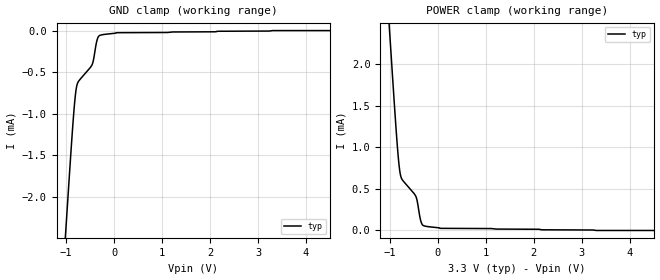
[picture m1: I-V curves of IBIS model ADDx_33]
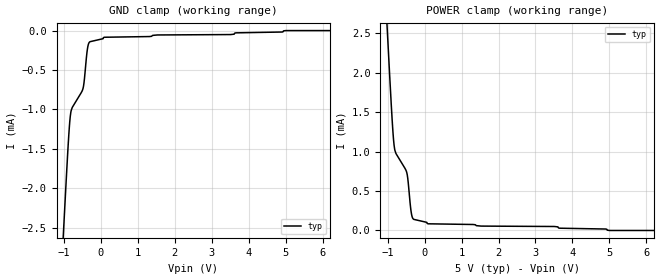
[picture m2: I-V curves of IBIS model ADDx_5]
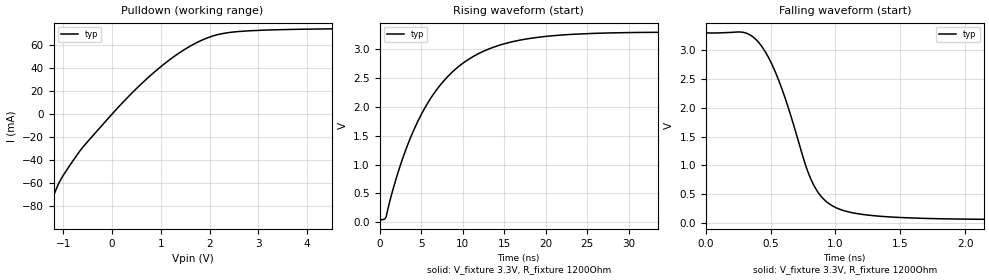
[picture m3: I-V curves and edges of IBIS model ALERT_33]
|Texas Instruments Incorporated
|Digital Temperature Sensor
|   with I2C Interface
| Marketing part#   Digital Voltage Range   Package-type   #pins
|TMP101NA/250   2.7 to 5.5   SOT   6
|TMP101NA/250G4   2.7 to 5.5   SOT   6
|TMP101NA/3K   2.7 to 5.5   SOT   6
|TMP101NA/3KG4   2.7 to 5.5   SOT   6
[IBIS Ver]   4.0
[File name]   tmp101.ibs
[File Rev]   1.0
[Date]   12/16/2010
[Source]   Texas Instruments Incorporated.
   Analog-eLab, HPA
   12500 TI Blvd
   Dallas, TX -75243
   For Support e-mail: elab_ibis@list.ti.com
[Notes]   Revision History:
   1.0: 12/16/2010
   - Model only contains nominal corner (27 degC, nominal
   process) for supply voltages of 3.3V and 5V.
   - Initial version of the model
   - Initial Model generated from simulations in TIspiceD
   - Model names with a trailing _33 contains the model for
   3.3V (3V and 3.6V). Model names with trailing _5 contains
   the model for 5V (4.5V and 5.5V) operation.
   - Model not matched to measurements
   - C_comp although listed in numerical order of value are
   obtained from varying PVT conditions. For PVT conditions
   for each specific value refer the buffer description under
   respective [Model]. IBIS model user is responsible for using
   appropriate C_comp to simulate for Signal Integrity.
[Disclaimer]
 This product is designed as an aid for customers of Texas Instruments.
 No warranties, either expressed or implied, with respect to this third
 party software (if any) or with respect to its fitness for any
 particular purpose is claimed by Texas Instruments or the author. The
 software (if any) is provided solely on an "as is" basis. The entire
 risk as to its quality and performance is with the customer
[Copyright] (C) Copyright 2010 Texas Instruments Incorporated.
   All rights reserved.
|   TMP101
[Component]   tmp101na
[Manufacturer] TI
[Package]
| variable   typ   min   max
R_pkg  9.17700E-02   8.39500E-02   1.02750E-01
L_pkg  2.62153E+00nH 1.83581E+00nH 3.14479E+00nH
C_pkg  2.92380E-01pF 2.61315E-01pF 3.29240E-01pF
[Pin] signal_name  model_name  R_pin  L_pin C_pin
1   SCL   SCL   0.08549  2.54106nH  0.29348pF
2   GND   GND   0.08549  2.53425nH  0.29238pF
3   ALERT  ALERT   0.10275  3.14479nH  0.32924pF
4   VP   POWER   0.09434  2.77778nH  0.32057pF
5   ADD0   ADDx   0.09489  2.96445nH  0.31618pF
6   SDA   SDA   0.08395  1.83581nH  0.10636pF
|   Model Selectors
[Model Selector]  ADDx
ADDx_33  3.3V digital input
ADDx_5  5V digital input
[Model Selector]  ALERT
ALERT_33  3.3V digital input
ALERT_5  5V digital input
[Model Selector]  SCL
SCL_33   3.3V digital input
SCL_5   5V digital input
[Model Selector]  SDA
SDA_33  3.3V digital I/O open-drain
SDA_5  5V digital I/O open-drain
[Model Selector]  TERM
TERM_33  3.3V anlaog buffers
TERM_5  5V analog buffers
|   TERM 3.3 V Model
[Model] TERM_33
Model_type Terminator
|   typ   min   max
C_comp   1.000e-200   NA   NA
[Voltage Range]   3.3   NA   NA
[Temperature Range]   27   NA   NA
|   TERM 5 V Model
[Model] TERM_5
Model_type Terminator
|   typ   min   max
C_comp   1.000e-200   NA   NA
[Voltage Range]   5   NA   NA
[Temperature Range]   27   NA   NA
| Models and submodels in the file (10): ADDx_33 (Input), ADDx_5 (Input), ALERT_33 (Open_drain), ALERT_5 (Open_drain), SCL_33 (Input), SCL_5 (Input), SDA_33 (I/O_open_drain), SDA_5 (I/O_open_drain), TERM_33 (Terminator), TERM_5 (Terminator)
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|   ADDx 3.3V Model
[Model]   ADDx_33
Model_type   Input
Vinl = 0.66
Vinh = 2.31
|   typ   min   max
C_comp   4.655pF   NA   NA
[Voltage Range]   3.3   NA   NA
[Temperature Range]   27   NA   NA
[Power Clamp Reference]   3.3   NA   NA
[GND Clamp Reference]   -0   NA   NA
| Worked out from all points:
|   GND clamp passes 1 mA (typ) near -0.84 V on its own axis
|   POWER clamp passes 1 mA (typ) near -0.84 V on its own axis
[GND Clamp]
|   Voltage   I(typ)   I(min)   I(max)
-3.3V     -16.09mA   NA         NA
-1.005V   -2.388mA   NA         NA
-866.1mV  -1.181mA   NA         NA
-819.7mV  -847.4uA   NA         NA
-789.3mV  -698.3uA   NA         NA
-740.5mV  -608.9uA   NA         NA
-462.8mV  -415.4uA   NA         NA
-432.6mV  -359.5uA   NA         NA
-354.5mV  -112.5uA   NA         NA
-301.5mV  -58.16uA   NA         NA
65.88mV   -25.49uA   NA         NA
6.59V     0A         NA         NA
[POWER Clamp]
|   Voltage   I(typ)   I(min)   I(max)
-3.3V     16.09mA    NA         NA
-1.005V   2.388mA    NA         NA
-866.1mV  1.181mA    NA         NA
-819.7mV  847.4uA    NA         NA
-789.3mV  698.3uA    NA         NA
-740.5mV  608.9uA    NA         NA
-462.8mV  415.4uA    NA         NA
-432.6mV  359.5uA    NA         NA
-354.5mV  112.5uA    NA         NA
-301.5mV  58.16uA    NA         NA
65.88mV   25.49uA    NA         NA
6.59V     0A         NA         NA
|   ADDx 5V Model
[Model]   ADDx_5
Model_type   Input
Vinl = 1.5
Vinh = 3.5
|   typ   min   max
C_comp   4.58pF   NA   NA
[Voltage Range]   5   NA   NA
[Temperature Range]   27   NA   NA
[Power Clamp Reference]   5   NA   NA
[GND Clamp Reference]   0   NA   NA
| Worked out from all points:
|   GND clamp passes 1 mA (typ) near -0.79 V on its own axis
|   POWER clamp passes 1 mA (typ) near -0.79 V on its own axis
[GND Clamp]
|   Voltage   I(typ)   I(min)   I(max)
-5V       -24.57mA   NA         NA
-1.059V   -2.977mA   NA         NA
-944mV    -1.951mA   NA         NA
-865.2mV  -1.304mA   NA         NA
-813mV    -1.037mA   NA         NA
-481.1mV  -730.8uA   NA         NA
-444.5mV  -611.3uA   NA         NA
-365.9mV  -239.7uA   NA         NA
-292.9mV  -140.9uA   NA         NA
98.01mV   -84.61uA   NA         NA
5.004V    0A         NA         NA
9.985V    0A         NA         NA
[POWER Clamp]
|   Voltage   I(typ)   I(min)   I(max)
-5V       24.57mA    NA         NA
-1.059V   2.977mA    NA         NA
-944mV    1.951mA    NA         NA
-865.2mV  1.304mA    NA         NA
-813mV    1.037mA    NA         NA
-481.1mV  730.8uA    NA         NA
-444.5mV  611.3uA    NA         NA
-365.9mV  239.7uA    NA         NA
-292.9mV  140.9uA    NA         NA
98.01mV   84.61uA    NA         NA
5.004V    0A         NA         NA
9.985V    0A         NA         NA
|   ALERT 3.3V Model
[Model]   ALERT_33
Model_type   Open_drain
Polarity   Non-Inverting
Enable   Active-Low
Vmeas = 1.65
Vref = 1.65
Cref = 15pF
Rref = 1200
|   typ   min   max
C_comp   5.68183e-12  NA   NA
|C_comp (ON state)   1.000e-200   NA   NA
|C_comp (OFF state)   1.000e-200   NA   NA
[Voltage Range]   3.3   NA   NA
[Temperature Range]   27   NA   NA
[Pullup Reference]   3.3   NA   NA
[Pulldown Reference]   0   NA   NA
[Power Clamp Reference]   3.3   NA   NA
[GND Clamp Reference]   0   NA   NA
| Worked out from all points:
|   slope of the pulldown table from 0 to 0.495 V, typ, clamps not added: 22.5 ohm
|   falling waveform, V_fixture 3.3V, R_fixture 1200Ohm: 20-80 % time 291ps typ, NA min, NA max; typ from 3.3 V to 0.058 V
|   rising waveform, V_fixture 3.3V, R_fixture 1200Ohm: 20-80 % time 7.23ns typ, NA min, NA max; typ from 0.058 V to 3.3 V
[Pulldown]
|   Voltage   I(typ)   I(min)   I(max)
-3.3V     -376.2mA   NA         NA
-1.388V   -96.12mA   NA         NA
-1.205V   -72mA      NA         NA
-1.082V   -59.25mA   NA         NA
-731.3mV  -36.24mA   NA         NA
-496.3mV  -23.69mA   NA         NA
263.5mV   12.04mA    NA         NA
852.5mV   35.94mA    NA         NA
1.381V    53.2mA     NA         NA
1.947V    66.06mA    NA         NA
2.797V    72.31mA    NA         NA
6.59V     75.64mA    NA         NA
[Ramp]
R_load = 1200
|   typ   min   max
dV/dt_r   1.94522/7.22568e-009 NA   NA
dV/dt_f   1.94527/2.91171e-010 NA   NA
[Falling Waveform]
V_fixture = 3.3V
R_fixture = 1200Ohm
C_fixture = 0F
|   Time   V(typ)   V(min)   V(max)
0s        3.3V       NA         NA
302.4ps   3.303V     NA         NA
432.2ps   3.065V     NA         NA
507.8ps   2.765V     NA         NA
588.1ps   2.322V     NA         NA
802.3ps   804mV      NA         NA
926.5ps   377.4mV    NA         NA
1.159ns   166.3mV    NA         NA
1.641ns   83.31mV    NA         NA
48.19ns   57.73mV    NA         NA
[Rising Waveform]
V_fixture = 3.3V
R_fixture = 1200Ohm
C_fixture = 0F
|   Time   V(typ)   V(min)   V(max)
0s        57.73mV    NA         NA
762.8ps   88.83mV    NA         NA
1.742ns   637.7mV    NA         NA
3.001ns   1.199V     NA         NA
5.819ns   2.074V     NA         NA
8.69ns    2.597V     NA         NA
12.3ns    2.952V     NA         NA
16.74ns   3.154V     NA         NA
22.05ns   3.248V     NA         NA
48.19ns   3.3V       NA         NA
